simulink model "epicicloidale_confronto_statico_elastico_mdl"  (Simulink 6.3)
settings: Solver=ode45  StartTime=0.0  StopTime=1  RelTol=1e-3
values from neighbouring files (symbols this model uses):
  b_c = kb*J_c    (= 4.94590955184)    [architetture_epicicloidale.m]    (also in architetture_epicicloidale_cont.m; architetture_epicicloidale_HEV.m = 92.8974810391; architetture_epicicloidale_prova.m; architetture_HEV_controllo.m = 9.28974810391)
  b_p = kb*J_p    (= 8.12277148259)    [architetture_epicicloidale_HEV.m]    (also in architetture_HEV_controllo.m = 0.812277148259; architetture_HEV_startstop.m = 0.0731049433433; Confronto_CVT_EMR.m = 0; epicicloidale_confronto_statico_elastico.m)
  b_r = kb*J_r    (= 218.026030555)    [architetture_epicicloidale.m]    (also in architetture_epicicloidale_cont.m; architetture_epicicloidale_HEV.m; architetture_epicicloidale_prova.m; architetture_HEV_controllo.m = 21.8026030555)
  b_s = kb*J_s    (= 8.12277148259)    [architetture_epicicloidale.m]    (also in architetture_epicicloidale_cont.m; architetture_epicicloidale_HEV.m = 4.94590955184; architetture_epicicloidale_prova.m; architetture_HEV_controllo.m = 0.494590955184)
  d_cr = d0    (= 10)    [architetture_epicicloidale_HEV.m]    (also in architetture_HEV_controllo.m = 1000; architetture_HEV_startstop.m = 90; epicicloidale_confronto_statico_elastico.m; epicicloidale_statico.m)
  d_sc = d0    (= 10)    [architetture_epicicloidale_HEV.m]    (also in architetture_HEV_controllo.m = 1000; architetture_HEV_startstop.m = 90; epicicloidale_confronto_statico_elastico.m; epicicloidale_statico.m)
  J_c = 1.3*0.5*pi*rho_acc*hc*r_c^4    (= 0.0494590955184)    [architetture_epicicloidale.m]    (also in architetture_epicicloidale_cont.m; architetture_epicicloidale_HEV.m = 0.928974810391; architetture_epicicloidale_prova.m; architetture_HEV_controllo.m = 0.928974810391)
  J_p = Nr_sat*0.5*pi*rho_acc*(hs*r_p^4 + hc*r_p^4)    (= 0.0812277148259)    [architetture_epicicloidale_HEV.m]    (also in architetture_HEV_controllo.m; architetture_HEV_startstop.m; Confronto_CVT_EMR.m = 0; epicicloidale_confronto_statico_elastico.m)
  J_r = 0.5*pi*rho_acc*(hr*r_ri^4 + h_ring*(r_re^4-r_ri^4))    (= 2.18026030555)    [architetture_epicicloidale.m]    (also in architetture_epicicloidale_cont.m; architetture_epicicloidale_HEV.m; architetture_epicicloidale_prova.m; architetture_HEV_controllo.m)
  J_s = Nr_sat*0.5*pi*rho_acc*(hs*r_s^4 + hc*r_s^4)    (= 0.0812277148259)    [architetture_epicicloidale.m]    (also in architetture_epicicloidale_cont.m; architetture_epicicloidale_HEV.m = 0.0494590955184; architetture_epicicloidale_prova.m; architetture_HEV_controllo.m = 0.0494590955184)
  K_cr = K0    (= 10000)    [architetture_epicicloidale_HEV.m]    (also in architetture_HEV_controllo.m = 100000; architetture_HEV_startstop.m = 10000000; epicicloidale_confronto_statico_elastico.m; epicicloidale_statico.m)
  K_sc = K0    (= 10000)    [architetture_epicicloidale_HEV.m]    (also in architetture_HEV_controllo.m = 100000; architetture_HEV_startstop.m = 10000000; epicicloidale_confronto_statico_elastico.m; epicicloidale_statico.m)
  Nr_sat = 4    [architetture_epicicloidale.m]    (also in architetture_epicicloidale_cont.m; architetture_epicicloidale_HEV.m; architetture_epicicloidale_prova.m; architetture_HEV_controllo.m)
  r_p = xds*Np/(2*pi)    (= 0.0732112738223)    [architetture_epicicloidale_HEV.m]    (also in architetture_HEV_controllo.m; architetture_HEV_startstop.m; Confronto_CVT_EMR.m = 0.025; epicicloidale_confronto_statico_elastico.m)
  r_r = xds*Nr/(2*pi)    (= 0.248281711223)    [architetture_epicicloidale_HEV.m]    (also in architetture_HEV_controllo.m; architetture_HEV_startstop.m; Confronto_CVT_EMR.m = 0.1; epicicloidale_confronto_statico_elastico.m)
  r_s = xds*Ns/(2*pi)    (= 0.0732112738223)    [architetture_epicicloidale.m]    (also in architetture_epicicloidale_cont.m; architetture_epicicloidale_HEV.m = 0.101859163579; architetture_epicicloidale_prova.m; architetture_HEV_controllo.m = 0.101859163579)
  Tau_c = 0*N*metri    (= 0)    [architetture_epicicloidale.m]    (also in architetture_epicicloidale_cont.m; architetture_epicicloidale_prova.m; epicicloidale.m; epicicloidale_confronto_statico_elastico.m = 10)
  Tau_r = 0*N*metri    (= 0)    [architetture_epicicloidale.m]    (also in architetture_epicicloidale_cont.m; architetture_epicicloidale_prova.m; epicicloidale.m; epicicloidale_confronto_statico_elastico.m = 20)
  Tau_s = 5*N*metri    (= 5)    [epicicloidale_confronto_statico_elastico.m]    (also in epicicloidale_statico.m = 0)
  Tc = 0.05*ms    (= 5e-05)    [architetture_epicicloidale.m]    (also in architetture_epicicloidale_cont.m; architetture_epicicloidale_HEV.m; architetture_epicicloidale_prova.m; architetture_HEV_controllo.m)
  Tc_0 = 0*N*metri    (= 0)    [architetture_epicicloidale_HEV.m]    (also in architetture_HEV_controllo.m; architetture_HEV_startstop.m; epicicloidale_confronto_statico_elastico.m; epicicloidale_statico.m)
  Tr_0 = 0*N*metri    (= 0)    [architetture_epicicloidale_HEV.m]    (also in architetture_HEV_controllo.m; architetture_HEV_startstop.m; epicicloidale_confronto_statico_elastico.m; epicicloidale_statico.m)
  Ts_0 = 0*N*metri    (= 0)    [architetture_epicicloidale_HEV.m]    (also in architetture_HEV_controllo.m; architetture_HEV_startstop.m; epicicloidale_confronto_statico_elastico.m; epicicloidale_statico.m)
  Wc_0 = 0*0.1*rad/secondo    (= 0)    [architetture_epicicloidale.m]    (also in architetture_epicicloidale_cont.m; architetture_epicicloidale_HEV.m; architetture_epicicloidale_prova.m; Confronto_CVT_EMR.m)
  Wr_0 = Sys1.C(3,:)*[Wc_0; Wsc_0]    [architetture_epicicloidale.m]    (also in Confronto_CVT_EMR.m = 0; epicicloidale.m; epicicloidale_confronto_statico_elastico.m = [-r_s/r_r, 1+r_s/r_r]*[Ws_0; Wc_0]; epicicloidale_da_solo.m = [ -1/r_ri*r_c, (r_c+r_ri)/r_ri]*[Wc_0; Wsc_0])
  Ws_0 = 0.1*rad/secondo    (= 0.1)    [epicicloidale_confronto_statico_elastico.m]    (also in epicicloidale_statico.m; architetture_epicicloidale_statico.m = 0)
undefined symbols (not defined in the file or in its folder): Wr, Ws
libraries: planetary_gear_blocks x2

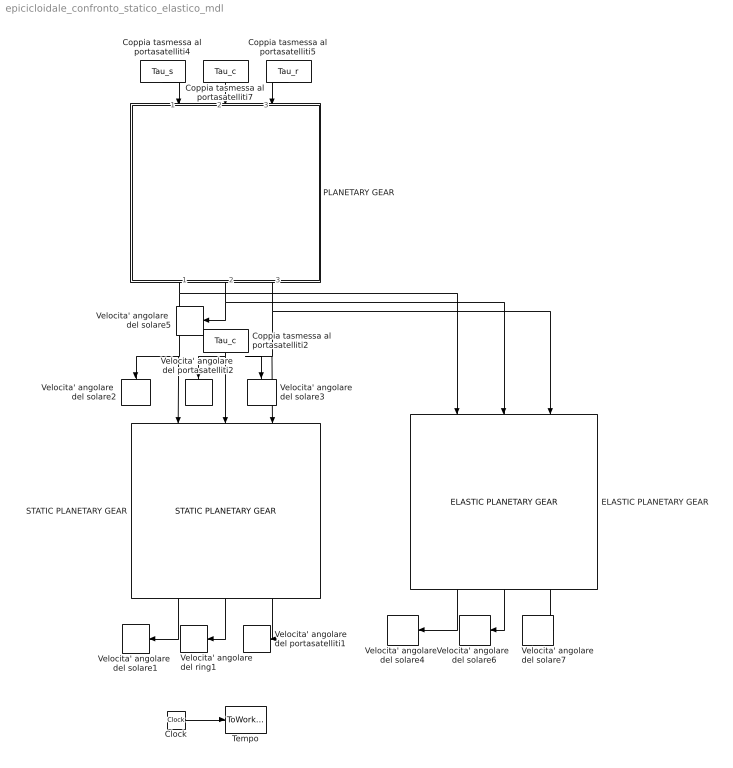
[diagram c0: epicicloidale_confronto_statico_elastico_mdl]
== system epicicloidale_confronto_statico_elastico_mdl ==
  Clock : Clock
  Coppia tasmessa al portasatelliti2 : Constant  Orientation=down  Value=Tau_c
  Coppia tasmessa al portasatelliti4 : Constant  Orientation=down  Value=Tau_s
  Coppia tasmessa al portasatelliti5 : Constant  Orientation=down  Value=Tau_r
  Coppia tasmessa al portasatelliti7 : Constant  Orientation=down  Value=Tau_c
  ELASTIC PLANETARY GEAR : planetary_gear_blocks/ELASTIC PLANETARY GEAR  Orientation=down  Par_solare=[J_s, b_s, r_s]  Par_satelliti=[J_p, J_c, b_p, b_c, r_p, Nr_sat]  Par_ring=[J_r, b_r, r_r]  Solare_Satelliti=[K_sc, d_sc]  Satelliti_Ring=[K_cr, d_cr]  Cond_in=[Ts_0, Tc_0, Tr_0]
  PLANETARY GEAR : Subsystem  Orientation=down  AncestorBlock=planetary_gear_blocks/PLANETARY GEAR  mask(POG Gruppo epicicloidale){Par_solare=[J_s, b_s, r_s], Par_satelliti=[J_p, J_c, b_p, b_c, r_p, Nr_sat], Par_ring=[J_r, b_r, r_r], Tipo_di_Modello=Modello esteso, Cond_in_Ws_Wc=[Ws_0,  Wc_0], Cond_in_Wc_Wr=[Wc_0,  Wr_0], Cond_in_Ws_Wr=[Ws_0,  Wr_0], Solare_Satelliti=[K_sc, d_sc], Satelliti_Ring=[K_cr, d_cr], Cond_in=[Ws_0, Wc_0, Wr_0]}
      mask prompts: Par_solare "Parametri Solare: [J_s, b_s, r_s]-->[kg*m^2,N*m*s/rad,m]"; Par_satelliti "Parametri Satelliti: [J_p, J_c, b_p, b_c, r_p, Nr_sat]-->[kg*m^2,N*m*s/rad,m]"; Par_ring "Parametri Ring: [J_r, b_r, r_r]-->[kg*m^2,N*m*s/rad,m,m]"; Tipo_di_Modello "Tipo di modello"; Cond_in_Ws_Wc "Condizioni iniziali: [Ws_0,  Wc_0]-->[rad/s]"; Cond_in_Wc_Wr "Condizioni iniziali: [Wc_0,  Wr_0]-->[rad/s]"; Cond_in_Ws_Wr "Condizioni iniziali: [Ws_0,  Wr_0]-->[rad/s]"; Solare_Satelliti "Solare-Satelliti: [K_sc, d_sc]-->[N/m,N*m*s/rad]"; Satelliti_Ring "Satelliti-Ring: [K_cr, d_cr]-->[N/m,N*m*s/rad]"; Cond_in "Condizioni iniziali: [Ws_0,  Wc_0, Wr_0]-->[rad/s]"
      mask help: Gruppo epicicloidale: [J_s, J_p, J_c, J_r]= Inerzie di: solare, satelliti, porta-satelliti, ring; [b_s, b_p, b_c, b_r]= Attriti di: solare, satelliti, porta-satelliti, ring; [r_s, r_p, r_r]= Raggi di: solare, satelliti, ring; [Nr_sat]= Numero Satelliti; [K_sc, K_cr]= Elasticita' tra solare-satelliti e tra satelliti-ring; [d_sc, d_cr]= Elementi della matrice D; [Ws_0, Wc_0, Wr_0]=Velocita' iniziali di solare, porta-satelliti, ring;
      mask init:
      | J_s=double(Par_solare(1));          
      | b_s=double(Par_solare(2));            
      | r_s=double(Par_solare(3));           
      | %
      | J_p=double(Par_satelliti(1));            
      | J_c=double(Par_satelliti(2));            
      | b_p=double(Par_satelliti(3));            
      | b_c=double(Par_satelliti(4));            
      | r_p=double(Par_satelliti(5));            
      | Nr_sat=double(Par_satelliti(6));           
      | %
      | J_r=double(Par_ring(1));             
      | b_r=double(Par_ring(2));            
      | r_r=double(Par_ring(3));                  
      | %
      | %%%%%%%%%%%%%%%%%%%%%%%%%%%%%%%%%%%%%%%%%%%%%%%%%%%%%%%%%%%%%%%%%%%%%%%%%%%
      | %   Modello esteso e modelli ridotti
      | %%%%%%%%%%%%%%%%%%%%%%%%%%%%%%%%%%%%%%%%%%%%%%%%%%%%%%%%%%%%%%%%%%%%%%%%%%%
      | if Tipo_di_Modello=='Modello esteso       '
      |     %
      |     K_sc=double(Solare_Satelliti(1));
      |     d_sc=double(Solare_Satelliti(2));
      |     if(K_sc==0)
      |         K_sc=inf;
      |     end
      |     %
      |     K_cr=double(Satelliti_Ring(1));
      |     d_cr=double(Satelliti_Ring(2));
      |     if(K_cr==0)
      |         K_cr=inf;
      |     end
      |     %
      |     %
      |     L=[ J_s,    0,      0,      0,      0,      0;
      |         0, 1/K_sc,      0,      0,      0,      0;
      |         0,      0,    J_p,      0,      0,      0;
      |         0,      0,      0,    J_c,      0,      0;
      |         0,      0,      0,      0, 1/K_cr,      0;
      |         0,      0,      0,      0,      0,    J_r];
      |     %
      |     A=- [-b_s-r_s^2*d_sc,                       -r_s,              -r_s*d_sc*r_p,                 r_s^2*d_sc,                          0,                          0;
      |                         r_s,                          0,                        r_p,                       -r_s,                          0,                          0;
      |               -r_s*d_sc*r_p,                       -r_p, -b_p-d_sc*r_p^2-d_cr*r_p^2,  r_s*d_sc*r_p-d_cr*r_p*r_r,                       -r_p,               d_cr*r_p*r_r;
      |                  r_s^2*d_sc,                        r_s,  r_s*d_sc*r_p-d_cr*r_p*r_r, -b_c-r_s^2*d_sc-d_cr*r_r^2,                       -r_r,                 d_cr*r_r^2;
      |                           0,                          0,                        r_p,                        r_r,                          0,                       -r_r;
      |                           0,                          0,               d_cr*r_p*r_r,                 d_cr*r_r^2,                        r_r,            -b_r-d_cr*r_r^2];
      | %                         
      |     B=[ 1, 0, 0;
      |         0, 0, 0;
      |         0, 0, 0;
      |         0, 1, 0;
      |         0, 0, 0;
      |         0, 0, 1];
      |     %
      |     C=[ 1, 0, 0, 0, 0, 0;
      |         0, 0, 0, 1, 0, 0;
      |         0, 0, 0, 0, 0, 1];
      |     %
      |     Ws_0=double(Cond_in(1));
      |     Wc_0=double(Cond_in(2));
      |     Wr_0=double(Cond_in(3));
      |     Wp_0=r_s*(Wc_0-Ws_0)/r_p;
      |     Wpc_0=[Wp_0 Wc_0];
      |     %
      |     We_0=[Ws_0 0 Wpc_0 0 Wr_0 ];
      |     %
      | elseif Tipo_di_Modello=='Modello ridotto Ws-Wc'
      |     L = [(J_s*r_p^2*r_r^2+r_s^2*J_p*r_r^2+r_s^2*J_r*r_p^2)/r_p^2/r_r^2,                                      -r_s*(r_s*J_p*r_r^2+J_r*r_p^2*r_s+J_r*r_p^2*r_r)/r_p^2/r_r^2;
      |            -r_s*(r_s*J_p*r_r^2+J_r*r_p^2*r_s+J_r*r_p^2*r_r)/r_p^2/r_r^2, (J_c*r_p^2*r_r^2+r_s^2*J_p*r_r^2+r_s^2*J_r*r_p^2+2*J_r*r_p^2*r_s*r_r+J_r*r_p^2*r_r^2)/r_p^2/r_r^2];
      |     %
      |     A=-[ -(b_s*r_p^2*r_r^2+r_s^2*b_p*r_r^2+r_s^2*b_r*r_p^2)/r_p^2/r_r^2,                                        r_s*(r_s*b_p*r_r^2+b_r*r_p^2*r_s+b_r*r_p^2*r_r)/r_p^2/r_r^2;
      |         r_s*(r_s*b_p*r_r^2+b_r*r_p^2*r_s+b_r*r_p^2*r_r)/r_p^2/r_r^2, -(b_c*r_p^2*r_r^2+r_s^2*b_p*r_r^2+r_s^2*b_r*r_p^2+2*b_r*r_p^2*r_s*r_r+b_r*r_p^2*r_r^2)/r_p^2/r_r^2];
      |     %
      |     B= [  1,             0,    -1/r_r*r_s;
      |            0,             1, (r_s+r_r)/r_r];
      |     %
      |     C= [            1,               0;
      |                     0,               1;
      |            -1/r_r*r_s, (r_s+r_r)/r_r];
      |     %
      |     Ws_0=double(Cond_in_Ws_Wc(1));
      |     Wc_0=double(Cond_in_Ws_Wc(2));
      |     We_0=[Ws_0 Wc_0];
      |     %
      | elseif Tipo_di_Modello=='Modello ridotto Wc-Wr'
      |     L= [ (J_c*r_s^2*r_p^2+J_s*r_p^2*r_s^2+2*J_s*r_p^2*r_s*r_r+J_s*r_p^2*r_r^2+r_r^2*J_p*r_s^2)/r_s^2/r_p^2,                                      -r_r*(J_s*r_p^2*r_s+J_s*r_p^2*r_r+r_r*J_p*r_s^2)/r_s^2/r_p^2;
      |           -r_r*(J_s*r_p^2*r_s+J_s*r_p^2*r_r+r_r*J_p*r_s^2)/r_s^2/r_p^2,                                     (J_r*r_s^2*r_p^2+J_s*r_p^2*r_r^2+r_r^2*J_p*r_s^2)/r_s^2/r_p^2];
      | 
      |     A=-[  -(b_c*r_s^2*r_p^2+b_s*r_p^2*r_s^2+2*b_s*r_p^2*r_s*r_r+b_s*r_p^2*r_r^2+r_r^2*b_p*r_s^2)/r_s^2/r_p^2,                                        r_r*(b_s*r_p^2*r_s+b_s*r_p^2*r_r+r_r*b_p*r_s^2)/r_s^2/r_p^2;
      |          r_r*(b_s*r_p^2*r_s+b_s*r_p^2*r_r+r_r*b_p*r_s^2)/r_s^2/r_p^2,                                     -(b_r*r_s^2*r_p^2+b_s*r_p^2*r_r^2+r_r^2*b_p*r_s^2)/r_s^2/r_p^2];
      | 
      |     B= [ (r_s+r_r)/r_s,    1,   0;
      |             -1/r_s*r_r,    0,   1];
      | 
      |     C= [ (r_s+r_r)/r_s,    -1/r_s*r_r;
      |                       1,            0;
      |                       0,            1];
      |     %
      |     Wc_0=double(Cond_in_Wc_Wr(1));
      |     Wr_0=double(Cond_in_Wc_Wr(2));
      |     We_0=[Wc_0 Wr_0];
      |     %
      | elseif Tipo_di_Modello=='Modello ridotto Ws-Wr'
      |     L= [ (J_c*r_s^2*r_p^2+J_s*r_p^2*r_s^2+2*J_s*r_p^2*r_s*r_r+J_s*r_p^2*r_r^2+r_r^2*J_p*r_s^2)/r_p^2/(r_s+r_r)^2,                                                      -r_s*r_r*(r_r*J_p*r_s-J_c*r_p^2)/r_p^2/(r_s+r_r)^2;
      |           -r_s*r_r*(r_r*J_p*r_s-J_c*r_p^2)/r_p^2/(r_s+r_r)^2, (J_r*r_s^2*r_p^2+2*J_r*r_p^2*r_s*r_r+J_r*r_p^2*r_r^2+r_r^2*J_p*r_s^2+r_r^2*J_c*r_p^2)/r_p^2/(r_s+r_r)^2];
      | 
      |     A=-[-(b_c*r_s^2*r_p^2+b_s*r_p^2*r_s^2+2*b_s*r_p^2*r_s*r_r+b_s*r_p^2*r_r^2+r_r^2*b_p*r_s^2)/r_p^2/(r_s+r_r)^2,                                                      -r_s*r_r*(-r_s*r_r*b_p+r_p^2*b_c)/r_p^2/(r_s+r_r)^2;
      |                                                               -r_s*r_r*(-r_s*r_r*b_p+r_p^2*b_c)/r_p^2/(r_s+r_r)^2, -(b_r*r_p^2*r_s^2+2*b_r*r_p^2*r_s*r_r+b_r*r_p^2*r_r^2+r_r^2*b_p*r_s^2+r_r^2*r_p^2*b_c)/r_p^2/(r_s+r_r)^2];
      | 
      |     B=[   1,  1/(r_s+r_r)*r_s, 0;
      |           0, 1/(r_s+r_r)*r_r, 1];
      | 
      |     C=[                 1,                  0;
      |          1/(r_s+r_r)*r_s, 1/(r_s+r_r)*r_r;
      |                         0,                  1];
      |     Ws_0=double(Cond_in_Ws_Wr(1));
      |     Wr_0=double(Cond_in_Ws_Wr(2));
      |     We_0=[Ws_0 Wr_0];
      | end
  STATIC PLANETARY GEAR : planetary_gear_blocks/STATIC PLANETARY GEAR  Orientation=down  Raggi_sun_ring=[r_s, r_r]  Tipo_di_Modello=Ws-Tc-Wr  Cond_in_Ws_Wc="[Ws_0,  Wc_0]"  Cond_in_Wc_Wr="[Wc_0,  Wr_0]"  Cond_in_Ws_Wr="[Ws_0,  Wr_0]"  Cond_in=[Ws_0, Wc_0, Wr_0]
  Tempo : ToWorkspace  VariableName=t  SampleTime=Tc  SaveFormat=Array
  Velocita' angolare del ring1 : ToWorkspace  VariableName=W  SampleTime=Tc  SaveFormat=Array
  Velocita' angolare  del portasatelliti1 : ToWorkspace  VariableName=Tau2  SampleTime=Tc  SaveFormat=Array
  Velocita' angolare  del portasatelliti2 : ToWorkspace  VariableName=Tau3  SampleTime=Tc  SaveFormat=Array
  Velocita' angolare  del solare1 : ToWorkspace  VariableName=Tau1  SampleTime=Tc  SaveFormat=Array
  Velocita' angolare  del solare2 : ToWorkspace  VariableName=W1  SampleTime=Tc  SaveFormat=Array
  Velocita' angolare  del solare3 : ToWorkspace  VariableName=W2  SampleTime=Tc  SaveFormat=Array
  Velocita' angolare  del solare4 : ToWorkspace  VariableName=Tau_s1  SampleTime=Tc  SaveFormat=Array
  Velocita' angolare  del solare5 : ToWorkspace  VariableName=W4  SampleTime=Tc  SaveFormat=Array
  Velocita' angolare  del solare6 : ToWorkspace  VariableName=Tau_c1  SampleTime=Tc  SaveFormat=Array
  Velocita' angolare  del solare7 : ToWorkspace  VariableName=Tau_r1  SampleTime=Tc  SaveFormat=Array
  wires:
  Clock/1 -> Tempo/1
  STATIC PLANETARY GEAR/1 -> Velocita' angolare  del solare1/1
  PLANETARY GEAR/1(Ws) -> Velocita' angolare  del solare2/1, STATIC PLANETARY GEAR/1, ELASTIC PLANETARY GEAR/1
  PLANETARY GEAR/2(Wc) -> Velocita' angolare  del solare5/1, ELASTIC PLANETARY GEAR/2
  PLANETARY GEAR/3(Wr) -> Velocita' angolare  del solare3/1, STATIC PLANETARY GEAR/3, ELASTIC PLANETARY GEAR/3
  Coppia tasmessa al portasatelliti2/1 -> Velocita' angolare  del portasatelliti2/1, STATIC PLANETARY GEAR/2
  Coppia tasmessa al portasatelliti4/1 -> PLANETARY GEAR/1(Ts)
  STATIC PLANETARY GEAR/2 -> Velocita' angolare del ring1/1
  STATIC PLANETARY GEAR/3 -> Velocita' angolare  del portasatelliti1/1
  ELASTIC PLANETARY GEAR/1 -> Velocita' angolare  del solare4/1
  ELASTIC PLANETARY GEAR/2 -> Velocita' angolare  del solare6/1
  ELASTIC PLANETARY GEAR/3 -> Velocita' angolare  del solare7/1
  Coppia tasmessa al portasatelliti5/1 -> PLANETARY GEAR/3(Tr)
  Coppia tasmessa al portasatelliti7/1 -> PLANETARY GEAR/2(Tc)

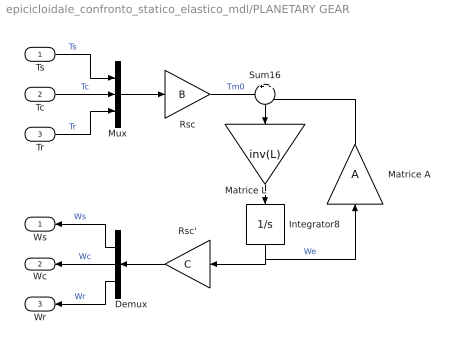
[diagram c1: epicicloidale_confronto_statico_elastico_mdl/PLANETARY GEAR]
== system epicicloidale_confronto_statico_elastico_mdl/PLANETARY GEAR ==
  Ts : Inport
  Tc : Inport  Port=2
  Tr : Inport  Port=3
  Demux : Demux  Orientation=left  Outputs=3
  Integrator8 : Integrator  Orientation=down  InitialCondition=We_0  LowerSaturationLimit=0
  Matrice A : Gain  Orientation=up  Gain=A  Multiplication=Matrix(K*u)
  Matrice L : Gain  Orientation=down  Gain=inv(L)  Multiplication=Matrix(K*u)
  Mux : Mux  Inputs=3
  Rsc : Gain  Gain=B  Multiplication=Matrix(K*u)
  Rsc' : Gain  Orientation=left  Gain=C  Multiplication=Matrix(K*u)
  Sum16 : Sum  Orientation=down  Inputs=+|-
  Ws : Outport  Orientation=left
  Wc : Outport  Orientation=left  Port=2
  Wr : Outport  Orientation=left  Port=3
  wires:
  Demux/3 -> Wr/1  "Wr"
  Demux/2 -> Wc/1  "Wc"
  Demux/1 -> Ws/1  "Ws"
  Rsc'/1 -> Demux/1
  Mux/1 -> Rsc/1
  Tr/1 -> Mux/3  "Tr"
  Tc/1 -> Mux/2  "Tc"
  Ts/1 -> Mux/1  "Ts"
  Matrice A/1 -> Sum16/2
  Integrator8/1 -> Rsc'/1, Matrice A/1  "We"
  Matrice L/1 -> Integrator8/1
  Sum16/1 -> Matrice L/1
  Rsc/1 -> Sum16/1  "Tm0"
